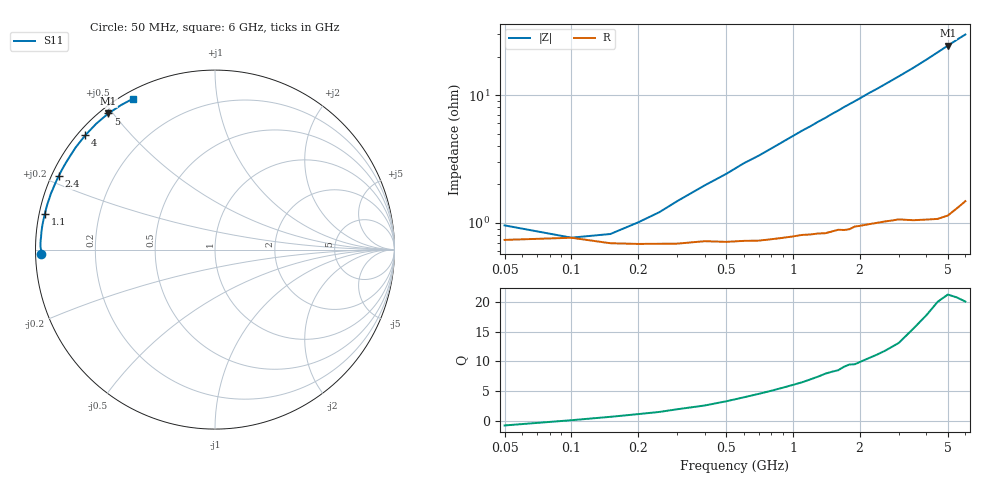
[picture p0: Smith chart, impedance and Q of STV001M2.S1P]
! SIEMENS Discrete & RF Semiconductors
! BA892
! Si PIN Diode in SCD-80
! IF = 1.2 mA
! S-Parameters:  September  1997
# GHz  S  MA  R  50
!  f  S11
! GHz  MAG  ANG
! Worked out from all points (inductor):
!   34 points, 50 MHz to 6 GHz, reference 50 ohm
!   read as one part to ground: L = 748 pH near 500 MHz
!   highest Q = 20.8 at 5 GHz (marker M1), where L = 774 pH
!   S11 on the Smith chart (normalised r, x): 50 MHz: 0.01, -0.01; 1.1 GHz: 0.02, +0.10; 2.4 GHz: 0.02, +0.22; 4 GHz: 0.02, +0.38; 5 GHz: 0.02, +0.49; 6 GHz: 0.03, +0.59
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0.05  0.9709 -178.6
0.1  0.9698 179.9
0.15  0.9726 179.0
0.2  0.9729 178.3
0.25  0.9729 177.7
0.3  0.9728 177.0
0.6  0.9715 173.5
0.7  0.9714 172.5
0.8  0.9707 171.4
1.1  0.9686 168.1
1.2  0.9684 167.1
1.3  0.9679 166.0
1.4  0.9678 165.0
1.5  0.9669 163.9
1.6  0.9659 162.9
1.7  0.9662 161.8
1.8  0.9658 160.8
2  0.964 158.8
2.2  0.9631 156.7
2.4  0.9625 154.8
2.8  0.9616 150.8
3  0.9612 148.8
3.5  0.9627 143.8
4  0.9635 138.6
4.5  0.9643 133.3
5  0.9637 128.1
5.5  0.9605 123.1
6  0.9572 118.5
